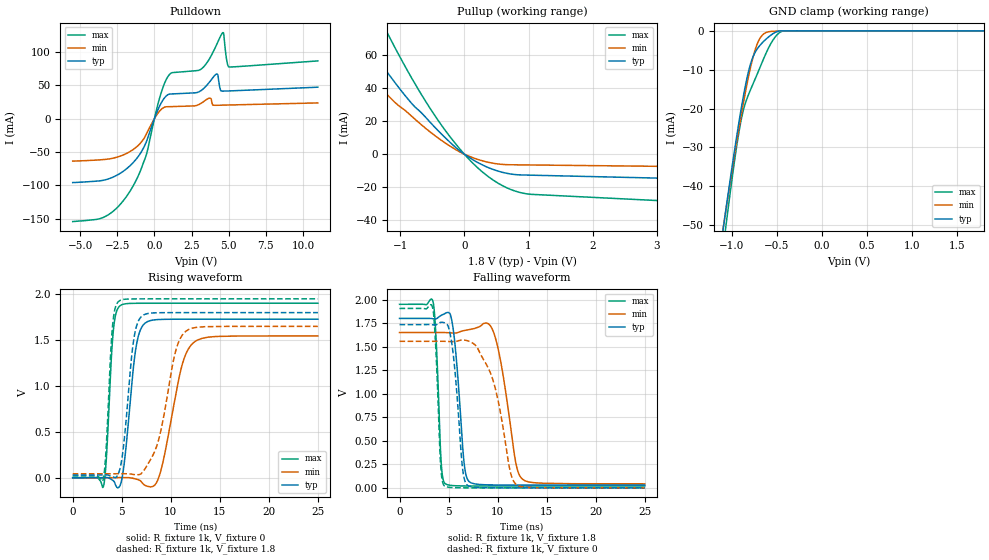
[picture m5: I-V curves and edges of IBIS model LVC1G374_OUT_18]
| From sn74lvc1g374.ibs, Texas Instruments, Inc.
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[Model]   LVC1G374_OUT_18
Model_type  3-state
Enable   Active-Low
Vref =   0
Rref =   1000
Cref =   30p
Vmeas =   0.9
| variable   typ   min   max
C_comp   5.62pF   4.86pF   6.45pF
| C_pullup   7.73pF   5.77pF   8.45pF
| C_pulldown   9.48pF   6.37pF   14.06pF
| C_tri-state   5.62pF   4.86pF   6.45pF
[Temperature Range]   40   100   -40
| Ambient temperature   25   85   -40
[Voltage range]   1.8   1.65   1.95
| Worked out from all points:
|   slope of the pulldown table from 0 to 0.27 V, typ, clamps not added: 18 ohm
|   slope of the pullup table from 0 to 0.27 V, typ, clamps not added: 42.8 ohm
|   GND clamp passes 1 mA (typ) near -0.56 V on its own axis
|   rising waveform, R_fixture 1k, V_fixture 0: 20-80 % time 954ps typ, 1.7ns min, 553ps max; typ from 0 V to 1.73 V
|   falling waveform, R_fixture 1k, V_fixture 1.8: 20-80 % time 752ps typ, 1.36ns min, 440ps max; typ from 1.8 V to 0.029 V
|   rising waveform, R_fixture 1k, V_fixture 1.8: 20-80 % time 921ps typ, 1.75ns min, 538ps max; typ from 0.029 V to 1.8 V
|   falling waveform, R_fixture 1k, V_fixture 0: 20-80 % time 790ps typ, 1.88ns min, 445ps max; typ from 1.74 V to 0 V
[GND Clamp]
| LVC1G374_OUT_18
|   Voltage   I(typ)   I(min)   I(max)
-5.5V     -897.8mA   -832.4mA   -1.016A
-1.11V    -52.82mA   -52.44mA   -57.96mA
-1.08V    -47.86mA   -47.85mA   -52.38mA
-1.05V    -42.97mA   -43.33mA   -46.9mA
-915mV    -22.35mA   -24.01mA   -24.95mA
-835mV    -12.29mA   -13.87mA   -17.5mA
-785mV    -7.843mA   -8.49mA    -14.64mA
-735mV    -5.197mA   -4.32mA    -11.95mA
-645mV    -2.635mA   -747.2uA   -6.981mA
-530mV    -538.4uA   -106uA     -1.891mA
-425mV    -4.773uA   -33.06uA   -14.75uA
1.8V      18.99pA    21.74nA    569.3pA
[Pulldown]
| LVC1G374_OUT_18
|   Voltage   I(typ)   I(min)   I(max)
-5.5V     -96.03mA   -63.8mA    -154.5mA
-3.47V    -92.68mA   -61.55mA   -148.6mA
-2.09V    -78.96mA   -54.47mA   -123.1mA
-605mV    -38mA      -26mA      -58.35mA
300mV     16.42mA    9.98mA     27.08mA
875mV     35.4mA     17.82mA    61.89mA
3.195V    42.96mA    23.74mA    75.16mA
3.745V    55.96mA    30.63mA    91.34mA
4.2V      66.99mA    20mA       111.6mA
4.6V      41.29mA    20.2mA     129mA
5.01V     41.55mA    20.42mA    77.37mA
11V       47.14mA    23.52mA    86.61mA
[Pullup]
| LVC1G374_OUT_18
|   Voltage   I(typ)   I(min)   I(max)
-5.5V     347.4mA    186.3mA    493.3mA
-2.1V     102.8mA    77.03mA    149.1mA
-1.685V   77.2mA     57.16mA    112.9mA
-1.265V   53.26mA    38.8mA     78.78mA
-1.185V   48.98mA    35.54mA    72.63mA
-865mV    32.91mA    24.65mA    49.37mA
-535mV    19.53mA    13.6mA     27.97mA
-10mV     279.4uA    182.4uA    442.5uA
225mV     -5.409mA   -3.38mA    -8.872mA
475mV     -9.653mA   -5.667mA   -16.4mA
950mV     -12.68mA   -6.523mA   -23.96mA
11V       -21.77mA   -10.67mA   -43.63mA
[Ramp]
| LVC1G374_OUT_18
| variable   typ   min   max
dV/dt_r   1.10/1.01E-09   0.99/1.80E-09   1.20/5.84E-10
dV/dt_f   1.10/7.90E-10   1.03/1.48E-09   1.19/4.64E-10
R_load = 1k
[Rising Waveform]
| LVC1G374_OUT_18
R_fixture =   1k
C_fixture =   0
L_fixture =   0
V_fixture =   0
V_fixture_min = 0
V_fixture_max = 0
|   Time   V(typ)   V(min)   V(max)
0s        121.3pV    6.876nV    2.208nV
3.14ns    1.978mV    -2.814uV   -92.52mV
4.12ns    -31.14mV   -164.4uV   1.578V
4.84ns    -82.2mV    1.772mV    1.876V
6.415ns   1.393V     -13.33mV   1.902V
7.37ns    1.685V     -83.18mV   1.902V
8.805ns   1.725V     12.39mV    1.902V
11.08ns   1.728V     1.2V       1.902V
12.31ns   1.728V     1.471V     1.902V
24.99ns   1.728V     1.546V     1.902V
[Falling Waveform]
| LVC1G374_OUT_18
R_fixture =   1k
C_fixture =   0
L_fixture =   0
V_fixture =   1.8
V_fixture_min = 1.65
V_fixture_max = 1.95
|   Time   V(typ)   V(min)   V(max)
0s        1.8V       1.65V      1.95V
3.415ns   1.797V     1.65V      1.977V
4.26ns    1.833V     1.65V      250.8mV
4.685ns   1.855V     1.65V      42.25mV
5.46ns    1.695V     1.645V     24.01mV
6.57ns    277.7mV    1.671V     20.34mV
7.115ns   64.72mV    1.681V     19.95mV
9.62ns    30.87mV    1.644V     19.62mV
12.52ns   29.51mV    93.08mV    19.6mV
24.99ns   29.37mV    42.63mV    19.6mV
[Rising Waveform]
| LVC1G374_OUT_18
R_fixture =   1k
C_fixture =   0
L_fixture =   0
V_fixture =   1.8
V_fixture_min = 1.65
V_fixture_max = 1.95
|   Time   V(typ)   V(min)   V(max)
0s        29.35mV    42.54mV    19.59mV
3.095ns   30.98mV    42.54mV    -25.61mV
4.045ns   9.786mV    42.45mV    1.635V
4.72ns    62.12mV    44.02mV    1.926V
6.205ns   1.493V     35.18mV    1.95V
7.08ns    1.764V     56.46mV    1.95V
8.645ns   1.799V     371.1mV    1.95V
10.43ns   1.8V       1.351V     1.95V
11.5ns    1.8V       1.594V     1.95V
24.99ns   1.8V       1.65V      1.95V
[Falling Waveform]
| LVC1G374_OUT_18
R_fixture =   1k
C_fixture =   0
L_fixture =   0
V_fixture =   0
V_fixture_min = 0
V_fixture_max = 0
|   Time   V(typ)   V(min)   V(max)
0s        1.735V     1.557V     1.906V
3.36ns    1.732V     1.557V     1.919V
4.2ns     1.758V     1.557V     231.5mV
4.6ns     1.753V     1.557V     19.04mV
5.36ns    1.514V     1.554V     3.249mV
6.405ns   226.6mV    1.571V     504.2uV
6.925ns   27.17mV    1.563V     232.8uV
9.445ns   625.7uV    1.172V     19.47uV
11.89ns   89.88uV    35.41mV    11.78uV
24.99ns   17.73uV    45.91uV    8.636uV
